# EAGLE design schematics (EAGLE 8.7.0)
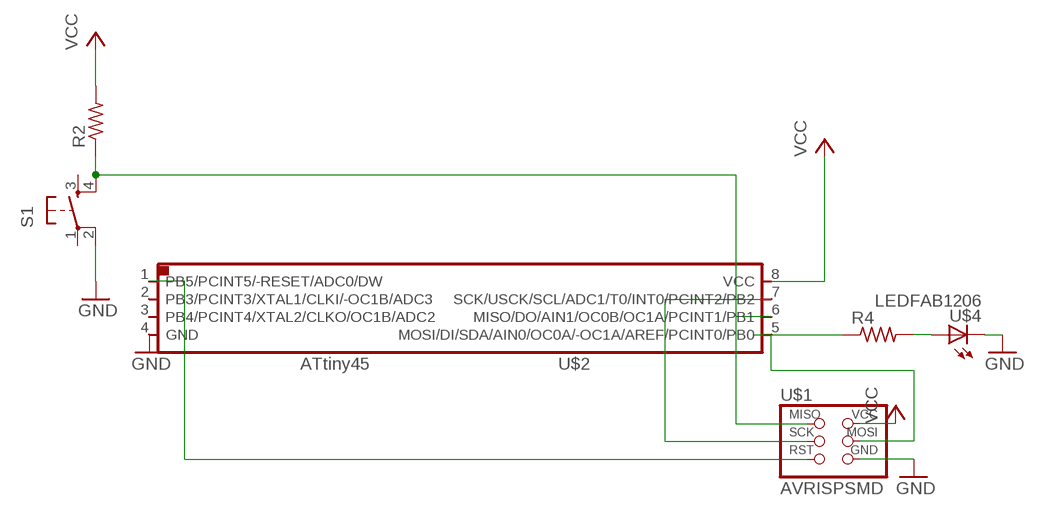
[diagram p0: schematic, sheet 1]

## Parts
R2  RES-US1206FAB  [R1206FAB]
R4  RES-US1206FAB  [R1206FAB]
S1  6MM_SWITCH6MM_SWITCH  [6MM_SWITCH]
U$1  AVRISPSMD  [2X03SMD]
U$2  ATTINY45SI  [SOIC8]
U$4  LEDFAB1206  [LED1206FAB]

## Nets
GND: S1.2(P1) U$1.6(GND) U$2.4(GND) U$4.2(C)
N$1: R4.1 U$1.4(MOSI) U$2.5(MOSI/DI/SDA/AIN0/OC0A/-OC1A/AREF/PCINT0/PB0)
N$2: R4.2 U$4.1(A)
N$3: R2.1 S1.4(S1) U$1.1(MISO) U$2.6(MISO/DO/AIN1/OC0B/OC1A/PCINT1/PB1)
N$10: U$1.5(RST) U$2.1(PB5/PCINT5/-RESET/ADC0/DW)
N$12: U$1.3(SCK) U$2.7(SCK/USCK/SCL/ADC1/T0/INT0/PCINT2/PB2)
VCC: R2.2 U$1.2(VCC) U$2.8(VCC)
Unconnected: S1.1(P) S1.3(S) U$2.2(PB3/PCINT3/XTAL1/CLKI/-OC1B/ADC3) U$2.3(PB4/PCINT4/XTAL2/CLKO/OC1B/ADC2)

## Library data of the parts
R2 R4 = fab:RES-US: Resistor (US Symbol)
S1 = fab:6MM_SWITCH: OMRON SWITCH
U$1 = fab:AVRISP
U$2 = fab:ATTINY45
U$4 = fab:LED: LED

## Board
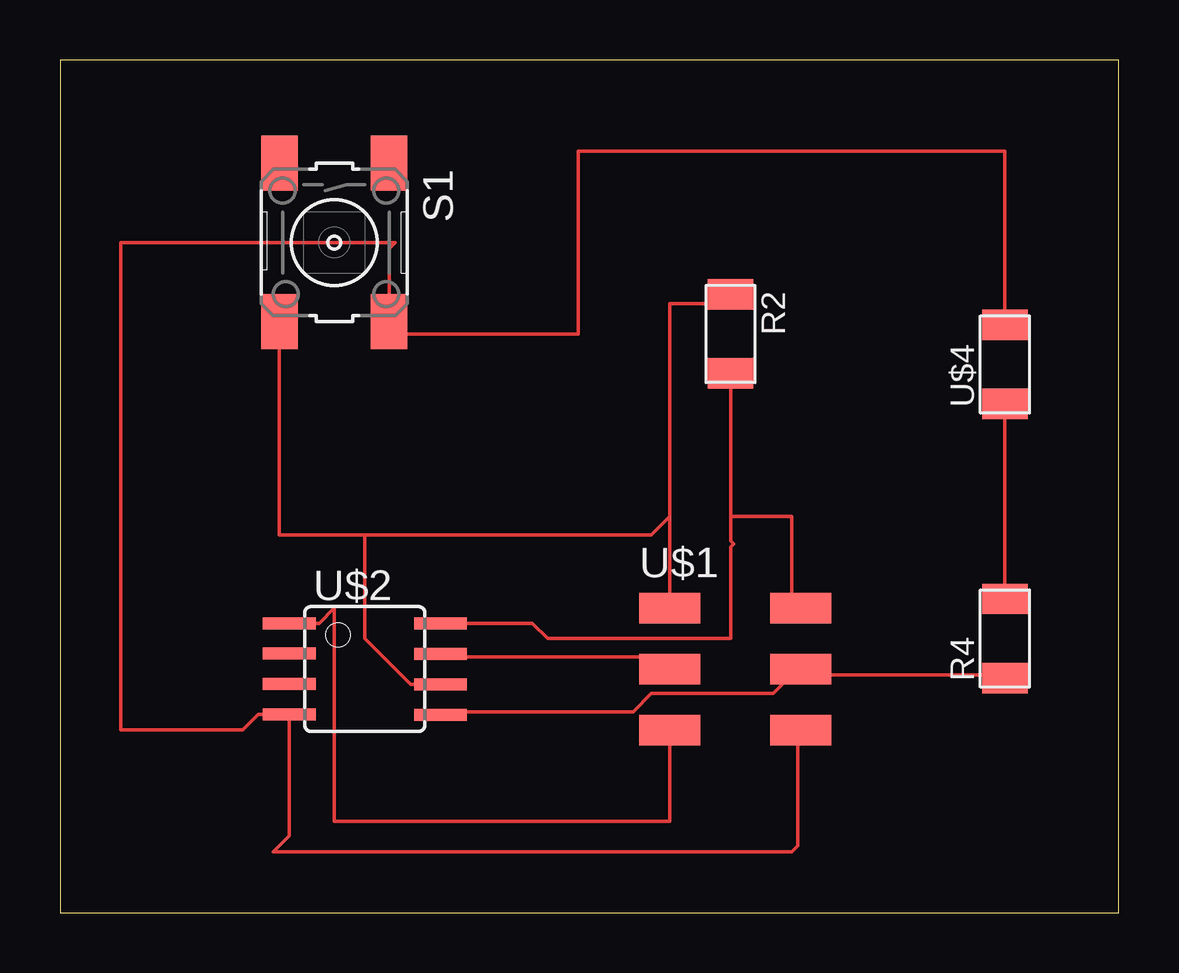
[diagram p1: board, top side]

Size 44.12 x 35.55 mm. Coordinates in mm from the lower left corner, seen from the top.
Outline: 0,0 44.12,0 44.12,35.55 0,35.55 0,0
Copper layers (1*16): Top 0.035mm / dielectric 1.5mm / Bottom 0.035mm
Design rules "default": minimum track width 6mil, minimum drill 0.35mm, track to track 6mil, track to pad 6mil, pad to pad 6mil, via to via 6mil, smd to smd 6mil, copper to edge 40mil, drill to drill 6mil, minimum pad ring 10mil, minimum via ring 8mil, stop-mask expansion 4mil, vias tented up to drill 0mil, thermal gap 10mil

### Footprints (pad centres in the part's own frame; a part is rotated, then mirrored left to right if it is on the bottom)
R1206FAB = smd 1.27 x 1.905: 1 -1.651,0; 2 1.651,0
6MM_SWITCH = smd 2.286 x 1.524: 1 -3.302,2.286; 2 3.302,2.286; 3 -3.302,-2.286; 4 3.302,-2.286
2X03SMD = smd 2.54 x 1.27: 1 -2.54,2.54; 2 2.92,2.54; 3 -2.54,0; 4 2.92,0; 5 -2.54,-2.54; 6 2.92,-2.54
SOIC8 = smd 0.5 x 2.2: 1 -1.905,-3.154; 2 -0.645,-3.154; 3 0.625,-3.154; 4 1.895,-3.154; 5 1.905,3.154; 6 0.635,3.154; 7 -0.635,3.154; 8 -1.905,3.154
LED1206FAB = smd 1.27 x 1.905: 1 -1.651,0; 2 1.651,0

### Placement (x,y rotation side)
R2  27.94,24.13 270 top
R4  39.37,11.43 90 top
S1  11.43,27.94 270 top
U$1  27.94,10.16 0 top
U$2  12.7,10.16 270 top
U$4  39.37,22.86 90 top

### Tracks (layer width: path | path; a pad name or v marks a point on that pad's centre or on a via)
GND
  Top 0.152: 9.65,8.13 U$2.4 | U$1.6 30.73,7.62 30.73,2.79 30.48,2.54 8.89,2.54 9.55,3.2 U$2.4 | 39.37,24.64 U$4.2 | 39.37,24.38 U$4.2 | U$2.4 8.27,8.27 7.62,7.62 2.54,7.62 2.54,27.94 13.97,27.94 13.72,27.69 S1.2 14.22,24.13 21.59,24.13 21.59,31.75 39.37,31.75 U$4.2
N$1
  Top 0.152: R4.1 39.37,9.91 31.24,9.91 30.99,10.16 U$1.4 30.73,10.16 29.72,9.14 24.64,9.14 23.88,8.38 16,8.38 U$2.5
N$2
  Top 0.152: U$4.1 R4.2
N$3
  Top 0.152: U$1.1 25.4,16.51 | 25.4,16.51 25.4,25.4 27.56,25.4 R2.1 | 15.24,9.65 15.75,9.65 U$2.6 14.61,9.53 12.7,11.43 12.7,15.75 | S1.4 9.14,15.75 12.7,15.75 | 12.7,15.75 24.64,15.75 25.4,16.51
N$10
  Top 0.152: 10.41,11.94 9.65,11.94 U$2.1 10.79,12.06 11.43,12.7 11.43,3.81 25.4,3.81 U$1.5
N$12
  Top 0.152: U$1.3 24.89,10.67 16,10.67 U$2.7
VCC
  Top 0.152: 27.94,22.61 R2.2 27.94,16.51 | 27.94,16.51 27.94,15.49 28.07,15.37 27.94,15.24 27.94,11.43 20.32,11.43 19.68,12.06 U$2.8 16,11.94 | 30.73,12.7 U$1.2 30.48,13.08 30.48,16.51 27.94,16.51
